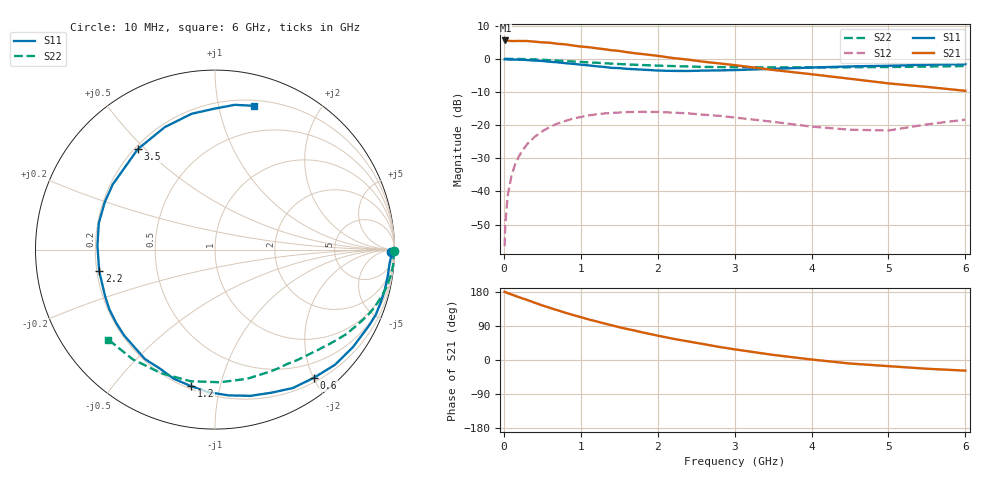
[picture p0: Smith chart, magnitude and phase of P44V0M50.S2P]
! SIEMENS Small Signal Semiconductors
! BFP182
! Si NPN RF Bipolar Junction Transistor in SOT143
! VCE = 4 V  IC = 0.5 mA
! Common Emitter S-Parameters:  March  1996
# GHz  S  MA  R  50
!  f  S11  S21  S12  S22
! GHz  MAG  ANG  MAG  ANG  MAG  ANG  MAG  ANG
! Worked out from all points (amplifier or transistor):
!   36 points, 10 MHz to 6 GHz, reference 50 ohm
!   highest |S21| = 5.5 dB at 20 MHz (marker M1)
!   |S21| within 3 dB of that: start of sweep to 1.421 GHz
!   unconditionally stable (mu >= 1): 2.95 GHz to end of sweep
!   at 250 MHz: K = 0.08, MSG = 16.4 dB, |S12| = -27.4 dB
!   at 1.4 GHz: K = 0.49, MSG = 9.4 dB, |S12| = -16.3 dB
!   at 6 GHz: K = 1.18, MAG = 1.8 dB, |S12| = -18.3 dB
!   S11 on the Smith chart (normalised r, x): 10 MHz: 63, -55; 600 MHz: 0.26, -2.01; 1.2 GHz: 0.22, -0.82; 2.2 GHz: 0.21, -0.09; 3.5 GHz: 0.21, +0.48; 6 GHz: 0.25, +1.28
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0.01  0.9821 -0.9  1.864 179.7  0.0015 85.7  0.999 -0.3
0.02  0.9838 -1.8  1.889 179.3  0.0034 85.5  0.9999 -0.6
0.05  0.9759 -4.3  1.876 176.5  0.0087 90.2  0.9974 -1.5
0.1  0.9738 -8.7  1.85 172.9  0.0174 83.4  0.9956 -3.1
0.15  0.9723 -13.5  1.851 169.2  0.0263 81.0  0.9964 -4.8
0.3  0.9567 -26.4  1.854 158.8  0.0511 73.0  0.9863 -9.4
0.4  0.9413 -35.2  1.811 151.2  0.0666 67.2  0.9779 -12.4
0.6  0.9021 -52.3  1.744 137.5  0.0941 56.3  0.9528 -18.1
0.8  0.8575 -68.3  1.649 124.7  0.1158 46.3  0.9253 -23.4
1.1  0.7956 -92.6  1.497 107.2  0.1398 33.0  0.8829 -30.2
1.2  0.7726 -99.9  1.443 102.1  0.1455 28.7  0.8722 -32.5
1.5  0.7241 -122.6  1.313 86.6  0.1549 18.1  0.834 -38.2
1.6  0.7053 -129.4  1.258 81.9  0.1573 15.0  0.8244 -39.9
1.9  0.6762 -150.6  1.143 68.7  0.1583 6.3  0.7973 -45.2
2.2  0.6564 -169.4  1.026 56.1  0.1543 -1.0  0.7763 -50.4
2.8  0.6686 156.8  0.852 34.5  0.1382 -12.2  0.7503 -61.3
3.5  0.7061 127.5  0.679 13.5  0.1122 -17.8  0.7418 -75.9
4  0.7374 112.3  0.585 1.3  0.095 -14.4  0.7397 -87.8
4.5  0.7679 99.7  0.5 -9.3  0.0853 -7.2  0.7458 -100.5
5  0.7856 90.1  0.426 -16.2  0.0831 7.6  0.7512 -113.5
5.5  0.8141 82.2  0.377 -23.1  0.1027 14.6  0.7641 -126.9
6  0.8297 74.9  0.329 -28.1  0.121 15.9  0.7773 -139.8
